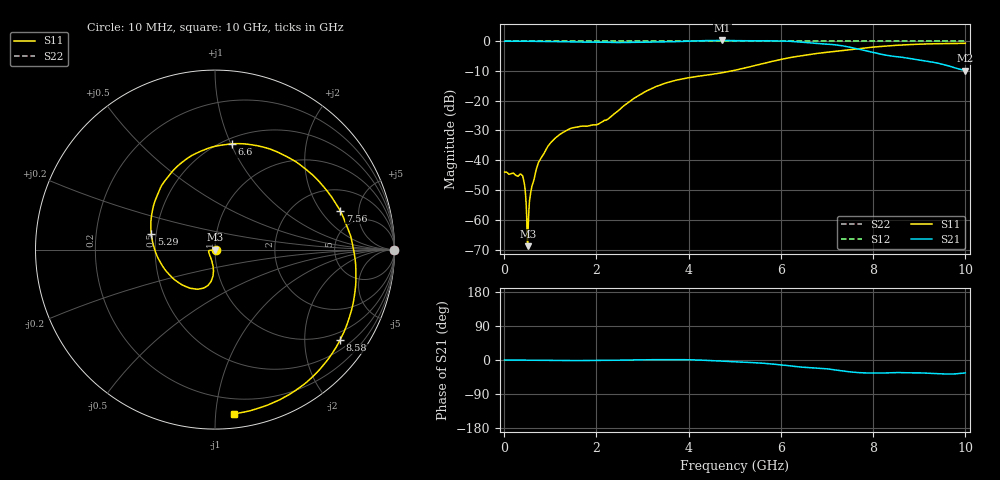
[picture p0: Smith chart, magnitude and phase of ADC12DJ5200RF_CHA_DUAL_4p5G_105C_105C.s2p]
! Texas Instruments, Inc.
! ADC12DJ5200RF - CH A S-Parameters (Dual Ch Mode, Fs = 4.5 GSPS, 105 degC case, 105 degC juntion)
! Port 1 represents the 100-ohm differenal input, Port 2 the digital output
! freq  dbS11  angS11  dbS21 angS21 dbS12 angS12 dbS22 angS22
# HZ S DB R 100
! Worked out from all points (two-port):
!   1000 points, 10 MHz to 10 GHz, reference 100 ohm
!   highest |S21| = 0.25 dB at 4.73 GHz (marker M1); lowest = -9.9 dB at 10 GHz (marker M2)
!   |S21| within 3 dB of the highest: start of sweep to 7.706 GHz
!   lowest |S11| = -68.9 dB at 510 MHz (marker M3), VSWR 1.00, Z = 100 - j0.0713 ohm
!   |S11| at or under -10 dB: start of sweep to 4.932 GHz
!   |S22| runs from 0.0 to 0.0 dB; largest |S21 - S12| = 0.76
!   S11 on the Smith chart (normalised r, x): 10 MHz: 1.01, -0.00; 5.29 GHz: 0.47, +0.10; 6.6 GHz: 0.55, +1.01; 7.56 GHz: 3.35, +3.13; 8.58 GHz: 0.75, -2.91; 10 GHz: 0.09, -1.12
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1e7  -43.98 -7.6  0.00 -0.0  0.00 0.0  0.00 0.0
3.8e8  -44.92 -10.5  0.01 -0.6  0.00 0.0  0.00 0.0
4.3e8  -47.24 -0.5  -0.00 -0.7  0.00 0.0  0.00 0.0
4.7e8  -52.81 6.8  -0.01 -0.7  0.00 0.0  0.00 0.0
5.1e8  -68.87 -81.6  -0.01 -0.8  0.00 0.0  0.00 0.0
6e8  -48.82 -136.8  -0.01 -0.9  0.00 0.0  0.00 0.0
7.1e8  -42.37 -157.4  -0.04 -0.9  0.00 0.0  0.00 0.0
9.4e8  -35.52 -169.1  -0.05 -1.3  0.00 0.0  0.00 0.0
1.26e9  -30.80 -171.7  -0.15 -1.7  0.00 0.0  0.00 0.0
1.68e9  -28.56 -163.4  -0.29 -1.5  0.00 0.0  0.00 0.0
2.24e9  -26.25 -119.8  -0.37 -1.2  0.00 0.0  0.00 0.0
3.34e9  -14.98 -96.9  -0.25 0.9  0.00 0.0  0.00 0.0
4.73e9  -10.59 -155.1  0.25 -3.1  0.00 0.0  0.00 0.0
5.01e9  -9.74 -174.4  0.20 -5.0  0.00 0.0  0.00 0.0
5.29e9  -8.74 165.9  0.14 -6.3  0.00 0.0  0.00 0.0
5.9e9  -6.49 126.2  0.11 -11.8  0.00 0.0  0.00 0.0
6.6e9  -4.49 81.1  -0.50 -19.9  0.00 0.0  0.00 0.0
6.67e9  -4.33 76.5  -0.60 -20.6  0.00 0.0  0.00 0.0
7.56e9  -2.73 17.4  -2.23 -32.1  0.00 0.0  0.00 0.0
8.34e9  -1.56 -25.8  -4.85 -33.9  0.00 0.0  0.00 0.0
8.58e9  -1.31 -35.9  -5.31 -33.2  0.00 0.0  0.00 0.0
1e10  -0.71 -83.2  -9.87 -34.1  0.00 0.0  0.00 0.0
